(* Logix 5000 AddOnInstructionDefinition export; software revision 16.04 *)

ADD_ON_INSTRUCTION AMCI_ANG1E_Immediate_Stop   (* revision 1.1, vendor AMCI *)
// Revision note:
// Version 1.1 added the slot_axis number and the input parameters can now be tags or discrete values.
VAR_INPUT
   slot_axis_number : INT; {required}
END_VAR
VAR_IN_OUT
   AMCI_ANG1E_output_data : INT[10]; {required}
END_VAR
VAR
   command_data_block : INT[10];
        [0]   // Command Bits MSW
        [1]   // Command Bits LSW
        [2]   // Upper Target Position
        [3]   // Lower Target Position
        [4]   // Upper Programmed Speed
        [5]   // Lower Programmed Speed
   index : INT;
END_VAR

ROUTINE Logic   (* ladder *)
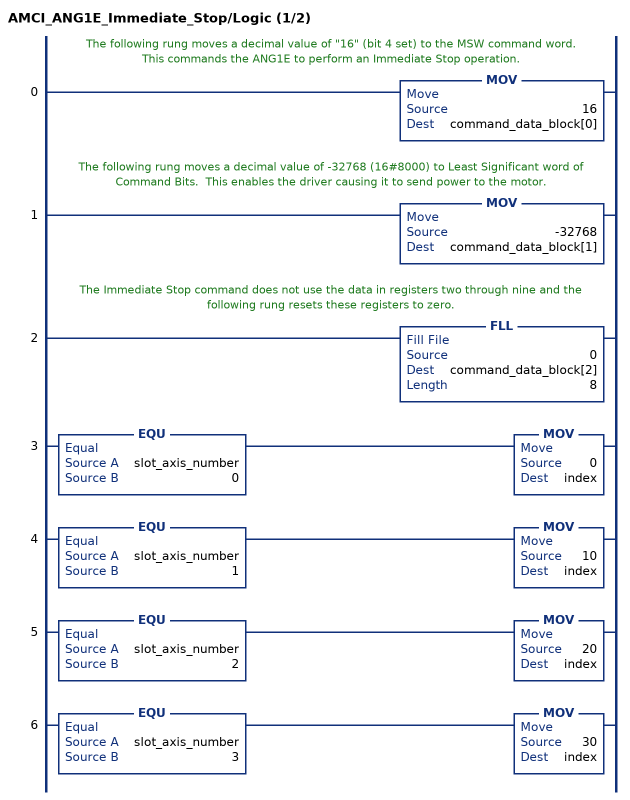
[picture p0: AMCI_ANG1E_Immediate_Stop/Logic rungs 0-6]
   // The following rung moves a decimal value of "16" (bit 4 set) to the MSW command word.  This commands the ANG1E to perform an Immediate Stop operation.
   0: MOV(16,command_data_block[0]);
   // The following rung moves a decimal value of -32768 (16#8000) to Least Significant word of Command Bits.  This enables the driver causing it to send power to the motor.
   1: MOV(-32768,command_data_block[1]);
   // The Immediate Stop command does not use the data in registers two through nine and the following rung resets these registers to zero.
   2: FLL(0,command_data_block[2],8);
   3: EQU(slot_axis_number,0)MOV(0,index);
   4: EQU(slot_axis_number,1)MOV(10,index);
   5: EQU(slot_axis_number,2)MOV(20,index);
   6: EQU(slot_axis_number,3)MOV(30,index);
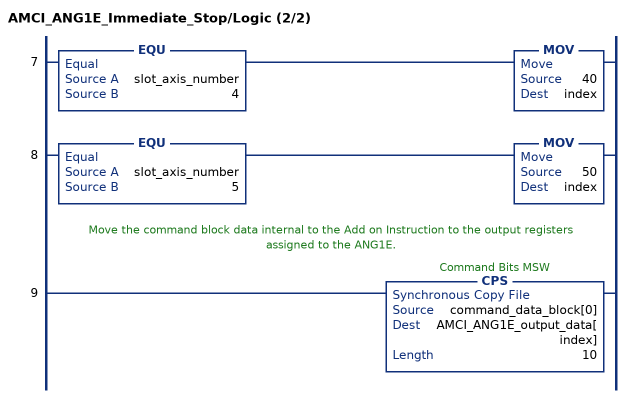
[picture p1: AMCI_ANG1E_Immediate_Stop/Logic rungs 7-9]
   7: EQU(slot_axis_number,4)MOV(40,index);
   8: EQU(slot_axis_number,5)MOV(50,index);
   // Move the command block data internal to the Add on Instruction to the output registers assigned to the ANG1E.
   9: CPS(command_data_block[0],AMCI_ANG1E_output_data[index],10);
END_ROUTINE
END_ADD_ON_INSTRUCTION
